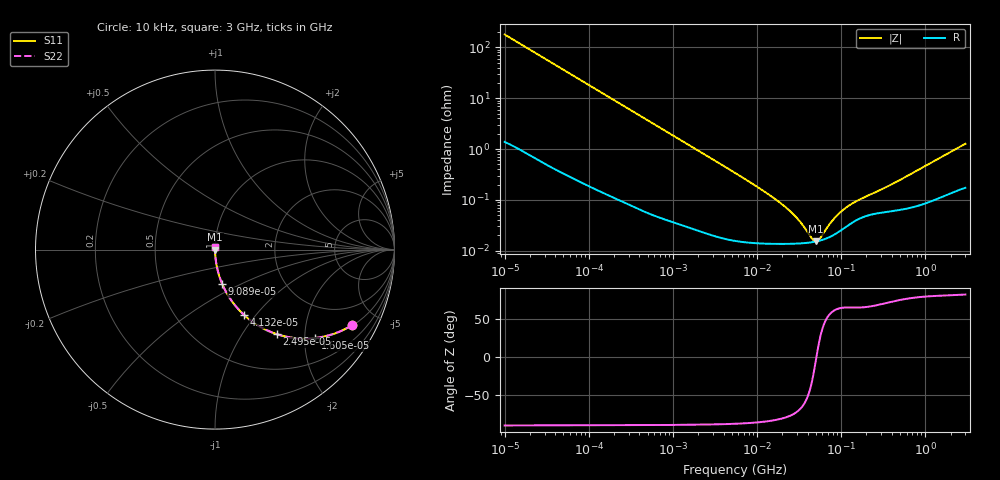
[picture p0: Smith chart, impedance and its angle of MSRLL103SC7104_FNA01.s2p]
! MSRLL103SC7104_FNA01  S-PARAMETER MODEL  ( Standard Model )
! Model Generated by TAIYO YUDEN Corporation (http://www.ty-top.com)
! Version 1.0
! TAIYO YUDEN Control No. 220601
! Copyright(c) 2010 TAIYO YUDEN CO.,LTD. All Rights Reserved.
! Product Description (link to TY-COMPAS)
! https://ds.yuden.co.jp/TYCOMPAS/or/detail?pn=MSRLL103SC7104MFNA01&u=M
! Products Name : Multilayer Ceramic Capacitors
! Characteristics :
!  Capacitance : 0.1 [uF] , Rated Voltage : 10 [V] , TCC : X7S
!  Case Size : 0.52 x 1.0 / 0.02 x 0.039 [mm/inch] , Thickness : 0.3 / 0.012 [mm/inch]
!  (Conditions: Temperature = 25 [degC] , DC Bias Voltage = 0 [V])
! External Node Assignments :
!  1  o---| |---o  2
! GND o---------o GND
! Frequency Range : 10kHz  -  3GHz  [ 401 STEP ]
# MHZ S RI R 50
! Freq[MHz].  S11 Real  S11 Imag  S21 Real  S21 Imag  S12 Real  S12 Imag  S22 Real  S22 Imag
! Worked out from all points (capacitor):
!   401 points, 10 kHz to 3 GHz, reference 50 ohm
!   read as one part in series: C = 88.2 nF near 10.65 kHz
!   lowest |Z| = 15.2 mohm at 49.78 MHz (marker M1)
!   series resonance near 50.84 MHz, so ESL is about 110 pH
!   S11 on the Smith chart (normalised r, x): 10 kHz: 1.03, -3.60; 16.05 kHz: 1.02, -2.25; 24.95 kHz: 1.01, -1.45; 41.32 kHz: 1.01, -0.88; 90.89 kHz: 1.00, -0.40; 3 GHz: 1.00, +0.03
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0.01  0.7626 -0.4216  0.2374 0.4216  0.2374 0.4216  0.7626 -0.4216
0.016047  0.5584 -0.4925  0.4416 0.4925  0.4416 0.4925  0.5584 -0.4925
0.024951  0.3462 -0.4716  0.6538 0.4716  0.6538 0.4716  0.3462 -0.4716
0.041322  0.1639 -0.3658  0.8361 0.3658  0.8361 0.3658  0.1639 -0.3658
0.056638  0.0956 -0.2895  0.9044 0.2895  0.9044 0.2895  0.0956 -0.2895
0.082683  0.0482 -0.2093  0.9518 0.2093  0.9518 0.2093  0.0482 -0.2093
0.090886  0.0405 -0.1921  0.9595 0.1921  0.9595 0.1921  0.0405 -0.1921
0.219733  0.00791 -0.0827  0.9921 0.0827  0.9921 0.0827  0.00791 -0.0827
0.683653  0.00118 -0.027  0.9988 0.027  0.9988 0.027  0.00118 -0.027
5.477226  0.000167 -0.0034  0.9998 0.0034  0.9998 0.0034  0.000167 -0.0034
12.83117  0.000139 -0.00138  0.9999 0.00138  0.9999 0.00138  0.000139 -0.00138
21.93027  0.000136 -0.000702  0.9999 0.000702  0.9999 0.000702  0.000136 -0.000702
32.0153  0.000139 -0.000358  0.9999 0.000358  0.9999 0.000358  0.000139 -0.000358
45.28751  0.000147 -8.69e-05  0.9999 8.69e-05  0.9999 8.69e-05  0.000147 -8.69e-05
49.78022  0.000151 -1.57e-05  0.9998 1.57e-05  0.9998 1.57e-05  0.000151 -1.57e-05
54.71863  0.000156 5.54e-05  0.9998 -5.54e-05  0.9998 -5.54e-05  0.000156 5.54e-05
79.88199  0.0002 0.000349  0.9998 -0.000349  0.9998 -0.000349  0.0002 0.000349
93.52181  0.000234 0.000476  0.9998 -0.000476  0.9998 -0.000476  0.000234 0.000476
112.9977  0.000291 0.000629  0.9997 -0.000629  0.9997 -0.000629  0.000291 0.000629
159.8419  0.000416 0.000895  0.9996 -0.000895  0.9996 -0.000895  0.000416 0.000895
374.4521  0.000592 0.00182  0.9994 -0.00182  0.9994 -0.00182  0.000592 0.00182
3000  0.00188 0.0125  0.9981 -0.0125  0.9981 -0.0125  0.00188 0.0125
